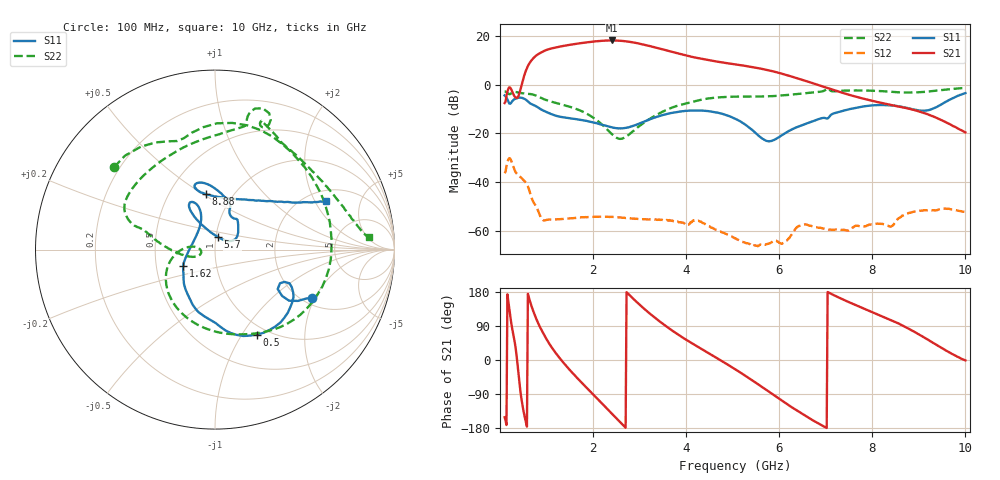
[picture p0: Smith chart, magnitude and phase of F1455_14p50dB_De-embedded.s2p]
! Integrated Device Technology
! Corporate Headquarters
! 6024 Silver Creek Valley Road
! San Jose, CA 95138  USA
! Phone:  1-408-284-8200
! Toll Free:  1-800-223-1366
! Webpage:  http://www.idt.com/
! Timing and RF Division
! 515 Groton Road, Suite 102
! Westford, MA 01886-6024
! Device:  F1455
! Description: 6-bit 0.5 dB Transmit Variable Gain Amplifier
! Frequency:  1400.0 -  2300.00 MHz
! Package:  6x6 mm Thin QFN Plastic Package: 28 pin
! State:  29
! Atten State:  14.5 dB
! Voltage:  +5.00 Volts
! Current:  217.643 mA
! Data:  The device was measured on a the F1455 evaluation board which has
!  individual transmission lines to the RF pins.  Data was collected
!  using a calibrated network analyzer.  The evaluation board was
!  de-embedded using a TRL calibration technique.
!  The reference plane is the edge of the package pin.
!  Pin  1 = CSb
!  Pin  2 = DATA
!  Pin  3 = CLK
!  Pin  4 = RSET
!  Pin  5 = GND
!  Pin  6 = RFIN  = Port 1
!  Pin  7 = GND
!  Pin  8 = NC
!  Pin  9 = NC
!  Pin 10 = NC
!  Pin 11 = NC
!  Pin 12 = NC
!  Pin 13 = NC
!  Pin 14 = /STBY
!  Pin 15 = GND
!  Pin 16 = RFOUT  = Port 2
!  Pin 17 = GND
!  Pin 18 = NC
!  Pin 19 = NC
!  Pin 20 = NC
!  Pin 21 = GND
!  Pin 22 = NC
!  Pin 23 = GND
!  Pin 24 = NC
!  Pin 25 = NC
!  Pin 26 = NC
!  Pin 27 = GND
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# GHz S dB R 50
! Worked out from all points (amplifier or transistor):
!   496 points, 100 MHz to 10 GHz, reference 50 ohm
!   highest |S21| = 18.2 dB at 2.4 GHz (marker M1)
!   |S21| within 3 dB of that: 1.171 GHz to 3.363 GHz (2.191 GHz wide, 96.7 % of centre)
!   unconditionally stable (mu >= 1): start of sweep to end of sweep
!   at 1.74 GHz: K = 32.39, MAG = 17.6 dB, |S12| = -54.4 dB
!   at 5.06 GHz: K = 174.85, MAG = 10.3 dB, |S12| = -63.0 dB
!   at 10 GHz: K = 275.35, MAG = -11.0 dB, |S12| = -52.3 dB
!   S11 on the Smith chart (normalised r, x): 100 MHz: 2.25, -1.90; 500 MHz: 0.89, -1.16; 1.62 GHz: 0.69, -0.13; 5.7 GHz: 1.02, +0.15; 8.88 GHz: 0.75, +0.52; 10 GHz: 2.47, +2.46
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0.1  -4.37 -26.4  -7.50 -151.1  -36.29 45.7  -2.78 140.8
0.24  -7.40 -24.9  -1.80 99.7  -31.10 -62.8  -3.56 101.3
0.38  -5.40 -41.0  -5.26 -14.5  -36.87 -114.6  -3.14 57.4
0.5  -5.56 -63.8  2.42 -131.0  -38.97 -153.1  -3.51 27.5
0.68  -7.96 -91.7  10.08 141.5  -46.40 143.1  -3.90 -14.3
0.82  -9.34 -109.6  12.55 97.3  -51.77 120.7  -4.80 -46.0
0.96  -10.86 -123.0  13.99 63.9  -55.67 124.2  -6.05 -71.3
1.28  -13.10 -142.3  15.64 5.6  -55.17 93.0  -7.84 -114.8
1.62  -14.06 -153.2  16.76 -42.4  -54.65 63.0  -9.80 -147.6
1.76  -14.47 -157.1  17.14 -60.4  -54.38 52.6  -10.88 -158.6
2.08  -15.80 -168.2  17.87 -100.6  -54.14 32.5  -14.53 -179.6
2.4  -17.47 171.2  18.19 -141.0  -54.25 15.0  -20.17 173.5
2.78  -17.37 135.4  17.64 171.6  -54.74 -1.5  -20.32 -159.7
3.08  -15.24 117.2  16.52 137.2  -55.16 -11.8  -15.73 -167.5
3.4  -13.01 111.0  14.99 104.8  -55.37 -21.9  -11.99 179.4
4.08  -10.62 115.6  11.64 47.5  -56.94 -36.8  -7.32 164.0
5.06  -13.96 121.5  8.36 -24.8  -63.02 -82.0  -4.87 148.6
5.7  -22.80 77.4  6.24 -77.1  -65.70 -63.8  -4.78 122.3
6.7  -15.14 42.3  0.78 -157.6  -58.02 -134.1  -3.20 78.5
8.36  -8.41 107.0  -8.18 107.2  -58.07 147.3  -2.82 62.4
8.88  -10.10 99.1  -10.26 76.1  -52.13 137.4  -3.18 41.9
10  -3.43 23.8  -19.55 -1.0  -52.34 59.5  -1.29 4.6
